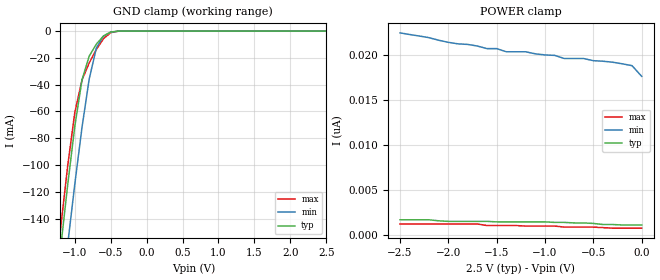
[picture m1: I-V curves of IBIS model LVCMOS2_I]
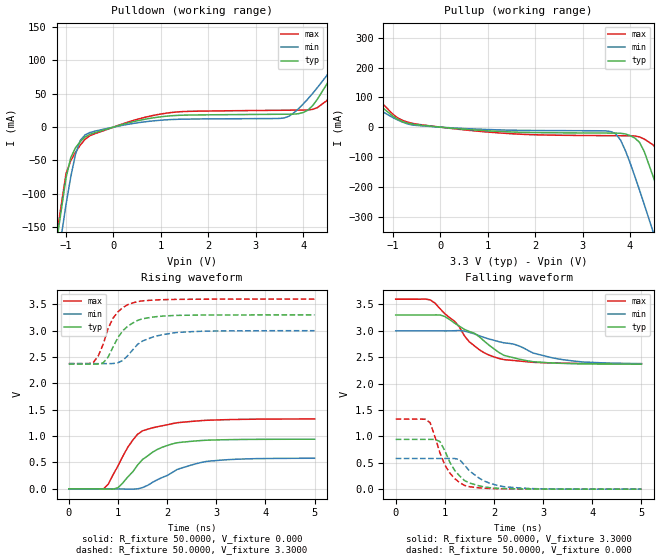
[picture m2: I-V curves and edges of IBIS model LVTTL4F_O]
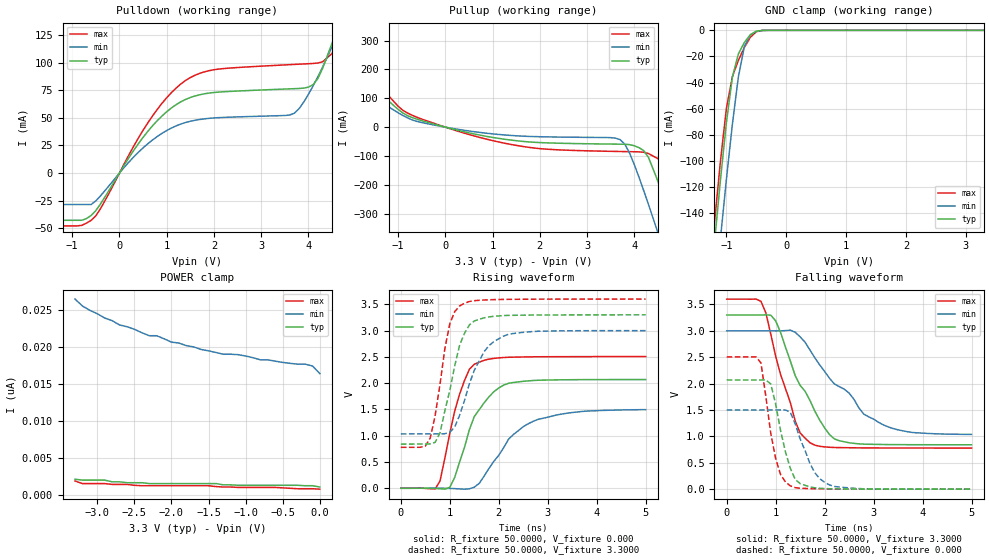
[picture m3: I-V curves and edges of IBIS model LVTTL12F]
| / 7\'7   Xilinx SpartanII I/O Buffer IBIS File
| \ \   Xilinx Inc.
| / /   2100 Logic Drive
| \_\/.\   San Jose,   CA 95124
[IBIS ver]   2.1
[File name]   spartan2.ibs
[File Rev]   1.5
[Date]   Apr. 26, 2002
[Source]   Hspice simulations (23e: TT, SS, FF)
[Notes]   Xilinx IBIS model for SpartanII I/O
   The package models are provided for VQ100, TQ144, CS144,
   PQ208, FG256 and FG456 package types, with VQ100 being
   selected as a default. Please make your own selection of
   the packages by commenting out the unused ones.
   COMMENTS: Models include process corners for MIN and MAX.
[Disclaimer] The data in this model is derived from SPICE simulations using
   modeling information extracted from the target process. While
   a great deal of care has been taken to provide information
   that is accurate, this model is considered preliminary as it
   has not been verified by actual silicon measurement. Treat the
   data in this model as preliminary until actual silicon
   verification is performed.
[Copyright]   Copyright 2000, Xilinx Inc., All rights reserved
|   Component Spartan-II
|   >>> Make Your Selection of the Package type Below <<<
[Component]   Spartan2
[Manufacturer]   Xilinx Inc.
[Package]
|--------------------------- XC2S15 -------------------------------
| XC2S15 with Package type VQ100:
| variable   typ   min   max
R_pkg   89.000m   83.000m   95.000m
L_pkg   4.5500nH   4.0000nH   5.1000nH
C_pkg   0.6500pF   0.6000pF   0.7000pF
| XC2S15 with Package type TQ144:
| variable   typ   min   max
|R_pkg   130.00m   123.00m   137.00m
|L_pkg   8.3500nH   7.5000nH   9.2000nH
|C_pkg   1.0500pF   0.8000pF   1.3000pF
| XC2S15 with Package type CS144:
| variable   typ   min   max
|R_pkg   109.50m   76.000m   143.00m
|L_pkg   2.2500nH   1.5000nH   3.0000nH
|C_pkg   0.2500pF   0.2000pF   0.3000pF
|--------------------------- XC2S30 -------------------------------
| XC2S30 with Package type VQ100:
| variable   typ   min   max
|R_pkg   84.500m   79.000m   90.000m
|L_pkg   4.3500nH   3.8000nH   4.9000nH
|C_pkg   0.6500pF   0.6000pF   0.7000pF
| XC2S30 with Package type TQ144:
| variable   typ   min   max
|R_pkg   130.00m   123.00m   137.00m
|L_pkg   8.3500nH   7.5000nH   9.2000nH
|C_pkg   1.0500pF   0.8000pF   1.3000pF
| XC2S30 with Package type CS144:
| variable   typ   min   max
|R_pkg   109.50m   76.000m   143.00m
|L_pkg   2.2500nH   1.5000nH   3.0000nH
|C_pkg   0.2500pF   0.2000pF   0.3000pF
| XC2S30 with Package type PQ208:
| variable   typ   min   max
|R_pkg   205.50m   205.00m   206.00m
|L_pkg   14.900nH   13.100nH   16.700nH
|C_pkg   1.9000pF   1.7000pF   2.1000pF
|--------------------------- XC2S50 -------------------------------
| XC2S50 with Package type TQ144:
| variable   typ   min   max
|R_pkg   123.50m   117.00m   130.00m
|L_pkg   7.9500nH   7.1000nH   8.8000nH
|C_pkg   1.0000pF   0.8000pF   1.2000pF
| XC2S50 with Package type PQ208:
| variable   typ   min   max
|R_pkg   195.50m   195.00m   196.00m
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[Pin]  signal_name   model_name   R_pin   L_pin   C_pin
1   LVCMOS2   LVCMOS2
1I   LVCMOS2_I   LVCMOS2_I
1O   LVCMOS2_O   LVCMOS2_O
2   LVTTL2F   LVTTL2F
2I   LVTTL2F_I   LVTTL2F_I
2O   LVTTL2F_O   LVTTL2F_O
3   LVTTL4F   LVTTL4F
3I   LVTTL4F_I   LVTTL4F_I
3O   LVTTL4F_O   LVTTL4F_O
4   LVTTL6F   LVTTL6F
4I   LVTTL6F_I   LVTTL6F_I
4O   LVTTL6F_O   LVTTL6F_O
5   LVTTL8F   LVTTL8F
5I   LVTTL8F_I   LVTTL8F_I
5O   LVTTL8F_O   LVTTL8F_O
6   LVTTL12F   LVTTL12F
6I   LVTTL12F_I   LVTTL12F_I
6O   LVTTL12F_O   LVTTL12F_O
7   LVTTL16F   LVTTL16F
7I   LVTTL16F_I   LVTTL16F_I
7O   LVTTL16F_O   LVTTL16F_O
8   LVTTL24F   LVTTL24F
8I   LVTTL24F_I   LVTTL24F_I
8O   LVTTL24F_O   LVTTL24F_O
9   LVTTL2S   LVTTL2S
9I   LVTTL2S_I   LVTTL2S_I
9O   LVTTL2S_O   LVTTL2S_O
10   LVTTL4S   LVTTL4S
10I   LVTTL4S_I   LVTTL4S_I
10O   LVTTL4S_O   LVTTL4S_O
11   LVTTL6S   LVTTL6S
11I   LVTTL6S_I   LVTTL6S_I
11O   LVTTL6S_O   LVTTL6S_O
12   LVTTL8S   LVTTL8S
12I   LVTTL8S_I   LVTTL8S_I
12O   LVTTL8S_O   LVTTL8S_O
13   LVTTL12S   LVTTL12S
13I   LVTTL12S_I   LVTTL12S_I
13O   LVTTL12S_O   LVTTL12S_O
14   LVTTL16S   LVTTL16S
14I   LVTTL16S_I   LVTTL16S_I
14O   LVTTL16S_O   LVTTL16S_O
15   LVTTL24S   LVTTL24S
15I   LVTTL24S_I   LVTTL24S_I
15O   LVTTL24S_O   LVTTL24S_O
16   HSTL1   HSTL1
16I   HSTL1_I   HSTL1_I
16O   HSTL1_O   HSTL1_O
17   HSTL3   HSTL3
17I   HSTL3_I   HSTL3_I
17O   HSTL3_O   HSTL3_O
18   HSTL4   HSTL4
18I   HSTL4_I   HSTL4_I
18O   HSTL4_O   HSTL4_O
19   SSTL2C1   SSTL2C1
19I   SSTL2C1_I   SSTL2C1_I
19O   SSTL2C1_O   SSTL2C1_O
20   SSTL2C2   SSTL2C2
20I   SSTL2C2_I   SSTL2C2_I
20O   SSTL2C2_O   SSTL2C2_O
21   SSTL3C1   SSTL3C1
21I   SSTL3C1_I   SSTL3C1_I
21O   SSTL3C1_O   SSTL3C1_O
22   SSTL3C2   SSTL3C2
22I   SSTL3C2_I   SSTL3C2_I
22O   SSTL3C2_O   SSTL3C2_O
23   CTT   CTT
23I   CTT_I   CTT_I
23O   CTT_O   CTT_O
24   AGP   AGP
24I   AGP_I   AGP_I
24O   AGP_O   AGP_O
25   GTL   GTL
25I   GTL_I   GTL_I
25O   GTL_O   GTL_O
26   GTL-PLUS   GTL-PLUS
26I   GTL-PLUS_I   GTL-PLUS_I
26O   GTL-PLUS_O   GTL-PLUS_O
27   PCI33M5V   PCI33M5V
27I   PCI33M5V_I   PCI33M5V_I
27O   PCI33M5V_O   PCI33M5V_O
28   PCI33M3V   PCI33M3V
28I   PCI33M3V_I   PCI33M3V_I
28O   PCI33M3V_O   PCI33M3V_O
29   PCI66M3V   PCI66M3V
29I   PCI66M3V_I   PCI66M3V_I
29O   PCI66M3V_O   PCI66M3V_O
PGND   GND   GND
VCCO   VCCO   POWER
| Models and submodels in the file (87): LVCMOS2 (I/O), LVCMOS2_I (Input), LVCMOS2_O (Output), LVTTL2F (I/O), LVTTL2F_I (Input), LVTTL2F_O (Output), LVTTL4F (I/O), LVTTL4F_I (Input), LVTTL4F_O (Output), LVTTL6F (I/O), LVTTL6F_I (Input), LVTTL6F_O (Output), LVTTL8F (I/O), LVTTL8F_I (Input), LVTTL8F_O (Output), LVTTL12F (I/O), LVTTL12F_I (Input), LVTTL12F_O (Output), LVTTL16F (I/O), LVTTL16F_I (Input), LVTTL16F_O (Output), LVTTL24F (I/O), LVTTL24F_I (Input), LVTTL24F_O (Output), LVTTL2S (I/O), LVTTL2S_I (Input), LVTTL2S_O (Output), LVTTL4S (I/O), LVTTL4S_I (Input), LVTTL4S_O (Output), LVTTL6S (I/O), LVTTL6S_I (Input), LVTTL6S_O (Output), LVTTL8S (I/O), LVTTL8S_I (Input), LVTTL8S_O (Output), LVTTL12S (I/O), LVTTL12S_I (Input), LVTTL12S_O (Output), LVTTL16S (I/O), LVTTL16S_I (Input), LVTTL16S_O (Output), LVTTL24S (I/O), LVTTL24S_I (Input), LVTTL24S_O (Output), HSTL1 (I/O), HSTL1_I (Input), HSTL1_O (Output), HSTL3 (I/O), HSTL3_I (Input), HSTL3_O (Output), HSTL4 (I/O), HSTL4_I (Input), HSTL4_O (Output), SSTL2C1 (I/O), SSTL2C1_I (Input), SSTL2C1_O (Output), SSTL2C2 (I/O), SSTL2C2_I (Input), SSTL2C2_O (Output), SSTL3C1 (I/O), SSTL3C1_I (Input), SSTL3C1_O (Output), SSTL3C2 (I/O), SSTL3C2_I (Input), SSTL3C2_O (Output), CTT (I/O), CTT_I (Input), CTT_O (Output), AGP (I/O), AGP_I (Input), AGP_O (Output), GTL (I/O_open_drain), GTL_I (Input), GTL_O (Open_drain), GTL-PLUS (I/O_open_drain), GTL-PLUS_I (Input), GTL-PLUS_O (Open_drain), PCI33M5V (I/O), PCI33M5V_I (Input)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
|   Model LVCMOS2_I
[Model]   LVCMOS2_I
Model_type   Input
Polarity   Non-Inverting
Vinl =   0.800V
Vinh =   1.700V
C_comp   6.5000pF   5.0000pF   8.0000pF
[Temperature Range]   27.0000   100.0000   0.000
[Voltage Range]   2.5000V   2.3750V   2.6250V
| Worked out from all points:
|   GND clamp passes 1 mA (typ) near -0.51 V on its own axis
[GND_clamp]
| voltage   I(typ)   I(min)   I(max)
-2.5V     -852.1mA   -861.3mA   -847.6mA
-1.2V     -163.3mA   -206.7mA   -148.3mA
-1.1V     -115.2mA   -159.6mA   -101mA
-1V       -71.03mA   -114.2mA   -60.76mA
-900mV    -36.42mA   -71.86mA   -36.51mA
-800mV    -18.71mA   -35.86mA   -23.83mA
-700mV    -9.708mA   -12.62mA   -13.62mA
-600mV    -3.604mA   -3.647mA   -5.596mA
-500mV    -691.4uA   -852.9uA   -1.154mA
-400mV    -68.33uA   -138.4uA   -98.29uA
2.5V      1.106nA    18.89nA    669.4pA
[POWER_clamp]
| voltage   I(typ)   I(min)   I(max)
-2.5V     1.688nA    22.47nA    1.222nA
-1.7V     1.513nA    21.01nA    1.222nA
-1.6V     1.513nA    20.72nA    1.048nA
-1.5V     1.455nA    20.72nA    1.048nA
-1.4V     1.455nA    20.37nA    1.048nA
-1.2V     1.455nA    20.37nA    989.5pA
-900mV    1.397nA    19.97nA    989.5pA
-800mV    1.397nA    19.62nA    873.1pA
-600mV    1.339nA    19.62nA    873.1pA
-200mV    1.106nA    19.03nA    756.7pA
-100mV    1.106nA    18.83nA    756.7pA
0V        1.106nA    17.64nA    756.7pA
|   Model LVTTL4F_O
[Model]   LVTTL4F_O
Model_type   Output
Polarity   Non-Inverting
Vmeas =   1.4000V
Cref =  35.0000pF
Rref =   1.0000M
Vref =  0.000V
C_comp   6.5000pF   5.0000pF   8.0000pF
[Temperature Range]   27.0000   100.0000   0.000
[Voltage Range]   3.3000V   3.0000V   3.6000V
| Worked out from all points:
|   slope of the pulldown table from 0 to 0.495 V, typ, clamps not added: 52.7 ohm
|   slope of the pullup table from 0 to 0.495 V, typ, clamps not added: 72 ohm
|   rising waveform, R_fixture 50.0000, V_fixture 0.000: 20-80 % time 649ps typ, 853ps min, 538ps max; typ from 0 V to 0.941 V
|   rising waveform, R_fixture 50.0000, V_fixture 3.3000: 20-80 % time 419ps typ, 526ps min, 353ps max; typ from 2.37 V to 3.3 V
|   falling waveform, R_fixture 50.0000, V_fixture 3.3000: 20-80 % time 914ps typ, 1.33ns min, 768ps max; typ from 3.3 V to 2.37 V
|   falling waveform, R_fixture 50.0000, V_fixture 0.000: 20-80 % time 386ps typ, 512ps min, 365ps max; typ from 0.943 V to 0.001 V
[Pulldown]
| voltage   I(typ)   I(min)   I(max)
-3.3V     -1.286A    -1.273A    -1.29A
-1.5V     -317.7mA   -354.1mA   -304.2mA
-1V       -76.21mA   -116mA     -69.81mA
-800mV    -30.95mA   -40.58mA   -37.74mA
-500mV    -10.89mA   -8.192mA   -12.96mA
1.2V      16.95mA    11.33mA    21.76mA
3.6V      19.37mA    13.78mA    25.36mA
4.1V      25.44mA    42.35mA    25.81mA
4.5V      64.6mA     77.61mA    39.82mA
5.1V      143.3mA    138.1mA    128.1mA
5.3V      171mA      159.5mA    161.3mA
6.6V      348mA      295mA      376.7mA
[Pullup]
| voltage   I(typ)   I(min)   I(max)
-3.3V     354.4mA    271.9mA    429.9mA
-2.7V     272.8mA    207.8mA    331mA
-800mV    18.43mA    17.03mA    23.04mA
3.6V      -19.96mA   -15.22mA   -28.65mA
3.8V      -20.52mA   -43.41mA   -28.84mA
4.2V      -51mA      -211.2mA   -32.92mA
4.5V      -171.4mA   -357.8mA   -61.08mA
4.7V      -272mA     -457.9mA   -116mA
4.9V      -376.2mA   -559mA     -210.3mA
5.1V      -482.2mA   -660.7mA   -313.6mA
5.3V      -589.2mA   -762.8mA   -420.3mA
6.6V      -1.293A    -1.432A    -1.133A
[Ramp]
| variable   typ   min   max
dV/dt_r   0.5647/0.6500n   0.3480/0.8497n   0.7950/0.5579n
dV/dt_f   0.5586/0.9517n   0.3726/1.3252n   0.7338/0.7688n
R_load = 50.0000
[Rising Waveform]
R_fixture = 50.0000
V_fixture = 0.000
| time   V(typ)   V(min)   V(max)
0s        0V         0V         0V
700ps     -2.021mV   226.2uV    -4.415mV
800ps     -4.588mV   188uV      85.45mV
1ns       21.52mV    -1.672mV   434.2mV
1.3ns     321.5mV    -6.047mV   921.4mV
1.5ns     557.2mV    23.94mV    1.1V
1.7ns     692mV      121.2mV    1.157V
2.2ns     873.5mV    365.6mV    1.253V
2.8ns     922.2mV    519.7mV    1.3V
5ns       941.2mV    580mV      1.325V
[Rising Waveform]
R_fixture = 50.0000
V_fixture = 3.3000
V_fixture_min = 3.0000
V_fixture_max = 3.6000
| time   V(typ)   V(min)   V(max)
0s        2.365V     2.374V     2.375V
500ps     2.365V     2.374V     2.397V
700ps     2.39V      2.374V     2.744V
800ps     2.499V     2.374V     3.043V
900ps     2.691V     2.377V     3.237V
1.1ns     3V         2.437V     3.439V
1.4ns     3.195V     2.74V      3.551V
1.7ns     3.256V     2.876V     3.579V
2.2ns     3.289V     2.966V     3.594V
5ns       3.299V     2.999V     3.599V
[Falling Waveform]
R_fixture = 50.0000
V_fixture = 3.3000
V_fixture_min = 3.0000
V_fixture_max = 3.6000
| time   V(typ)   V(min)   V(max)
0s        3.3V       3V         3.6V
700ps     3.299V     3V         3.587V
1ns       3.272V     2.999V     3.325V
1.2ns     3.145V     3.002V     3.18V
1.5ns     2.987V     2.97V      2.789V
1.8ns     2.807V     2.874V     2.584V
2.1ns     2.591V     2.795V     2.477V
2.7ns     2.429V     2.625V     2.411V
3.4ns     2.384V     2.454V     2.388V
5ns       2.369V     2.379V     2.377V
[Falling Waveform]
R_fixture = 50.0000
V_fixture = 0.000
| time   V(typ)   V(min)   V(max)
0s        943.3mV    581.6mV    1.327V
600ps     943.4mV    581.6mV    1.325V
700ps     943.7mV    581.6mV    1.262V
900ps     903.3mV    581.6mV    689.3mV
1ns       728.3mV    581.8mV    460.1mV
1.2ns     357.9mV    581.3mV    201.4mV
1.4ns     164mV      456.6mV    71.6mV
1.8ns     43.47mV    155.2mV    18.74mV
2.2ns     11.27mV    47.74mV    7.191mV
5ns       636.3uV    446.4uV    717.8uV
|   Model LVTTL12F
[Model]   LVTTL12F
Model_type   I/O
Polarity   Non-Inverting
Enable   Active-Low
Vinl =   0.800V
Vinh =   2.000V
Vmeas =   1.4000V
Cref =  35.0000pF
Rref =   1.0000M
Vref =  0.000V
C_comp   6.5000pF   5.0000pF   8.0000pF
[Temperature Range]   27.0000   100.0000   0.000
[Voltage Range]   3.3000V   3.0000V   3.6000V
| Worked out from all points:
|   slope of the pulldown table from 0 to 0.495 V, typ, clamps not added: 15.4 ohm
|   slope of the pullup table from 0 to 0.495 V, typ, clamps not added: 25.2 ohm
|   GND clamp passes 1 mA (typ) near -0.51 V on its own axis
|   rising waveform, R_fixture 50.0000, V_fixture 0.000: 20-80 % time 556ps typ, 797ps min, 400ps max; typ from 0 V to 2.07 V
|   rising waveform, R_fixture 50.0000, V_fixture 3.3000: 20-80 % time 372ps typ, 492ps min, 288ps max; typ from 0.84 V to 3.3 V
|   falling waveform, R_fixture 50.0000, V_fixture 3.3000: 20-80 % time 727ps typ, 1.07ns min, 508ps max; typ from 3.3 V to 0.841 V
|   falling waveform, R_fixture 50.0000, V_fixture 0.000: 20-80 % time 305ps typ, 397ps min, 266ps max; typ from 2.07 V to 0 V
[Pulldown]
| voltage   I(typ)   I(min)   I(max)
-3.3V     -42.8mA    -28.54mA   -47.89mA
-900mV    -42.8mA    -28.54mA   -47.89mA
-600mV    -38.47mA   -28.54mA   -42.9mA
700mV     42.79mA    29.97mA    51.76mA
1.2V      61.98mA    42.74mA    77.02mA
1.6V      69.81mA    47.81mA    88.61mA
3.7V      76.41mA    54.11mA    98.37mA
4.1V      80.11mA    79.08mA    99.25mA
4.3V      94.94mA    96.03mA    100.8mA
4.5V      117.6mA    114.4mA    108.3mA
4.7V      142.5mA    133.7mA    132.4mA
6.6V      399mA      330.4mA    441.4mA
[Pullup]
| voltage   I(typ)   I(min)   I(max)
-3.3V     401.3mA    308.2mA    484mA
-2.9V     344.8mA    263.9mA    415.5mA
-2.5V     286.5mA    217.5mA    345.7mA
-700mV    33.24mA    24.98mA    41.08mA
1.5V      -47.01mA   -30.01mA   -63.27mA
3.7V      -59.11mA   -43.28mA   -84.54mA
3.9V      -60.68mA   -90.11mA   -85.1mA
4.2V      -81.62mA   -220.4mA   -87.14mA
4.5V      -188mA     -366.4mA   -109.3mA
4.9V      -390.3mA   -567.4mA   -234.7mA
5.1V      -496.1mA   -669.1mA   -335.2mA
6.6V      -1.307A    -1.441A    -1.153A
[GND_clamp]
| voltage   I(typ)   I(min)   I(max)
-3.3V     -1.286A    -1.273A    -1.29A
-1.3V     -213.2mA   -255.1mA   -198mA
-1.2V     -163mA     -206.8mA   -147.7mA
-1.1V     -114.8mA   -159.6mA   -100.3mA
-1V       -70.57mA   -114.1mA   -59.86mA
-900mV    -35.79mA   -71.75mA   -35.46mA
-800mV    -18.04mA   -35.69mA   -22.98mA
-700mV    -9.256mA   -12.38mA   -13.06mA
-600mV    -3.388mA   -3.468mA   -5.299mA
-500mV    -637.4uA   -792.4uA   -1.07mA
-300mV    -3.973uA   -15.32uA   -4.185uA
3.3V      1.106nA    17.64nA    698.5pA
[POWER_clamp]
| voltage   I(typ)   I(min)   I(max)
-3.3V     2.095nA    26.43nA    1.863nA
-3.2V     1.979nA    25.49nA    1.513nA
-2.9V     1.979nA    23.87nA    1.513nA
-2.3V     1.513nA    21.48nA    1.222nA
-2.2V     1.513nA    21.48nA    1.222nA
-2V       1.513nA    20.61nA    1.222nA
-1.3V     1.339nA    18.98nA    1.048nA
-1.1V     1.281nA    18.92nA    989.5pA
-800mV    1.281nA    18.22nA    989.5pA
-200mV    1.222nA    17.64nA    814.9pA
-100mV    1.222nA    17.4nA     814.9pA
0V        1.048nA    16.36nA    756.7pA
[Ramp]
| variable   typ   min   max
dV/dt_r   1.2408/0.5535n   0.8970/0.7922n   1.5030/0.3954n
dV/dt_f   1.4752/0.7257n   1.1772/1.1183n   1.6925/0.5243n
R_load = 50.0000
[Rising Waveform]
R_fixture = 50.0000
V_fixture = 0.000
| time   V(typ)   V(min)   V(max)
0s        0V         0V         0V
700ps     -3.771mV   692.4uV    -13.4mV
800ps     -9.635mV   799.2uV    138.3mV
1ns       17.96mV    -3.585mV   1.048V
1.2ns     500.5mV    -12.31mV   1.792V
1.5ns     1.364V     21.02mV    2.359V
2ns       1.907V     627.7mV    2.48V
2.2ns     1.998V     933.5mV    2.492V
2.7ns     2.05V      1.273V     2.5V
5ns       2.068V     1.495V     2.505V
[Rising Waveform]
R_fixture = 50.0000
V_fixture = 3.3000
V_fixture_min = 3.0000
V_fixture_max = 3.6000
| time   V(typ)   V(min)   V(max)
0s        840.3mV    1.034V     778.4mV
500ps     841.4mV    1.034V     801.3mV
600ps     844.4mV    1.034V     955.5mV
800ps     1.055V     1.034V     1.98V
1ns       1.861V     1.067V     3.131V
1.2ns     2.721V     1.388V     3.467V
1.4ns     3.108V     1.987V     3.553V
1.7ns     3.242V     2.598V     3.582V
2.1ns     3.285V     2.895V     3.592V
5ns       3.299V     2.998V     3.599V
[Falling Waveform]
R_fixture = 50.0000
V_fixture = 3.3000
V_fixture_min = 3.0000
V_fixture_max = 3.6000
| time   V(typ)   V(min)   V(max)
0s        3.3V       3V         3.6V
700ps     3.299V     3V         3.558V
800ps     3.303V     3V         3.341V
1ns       3.19V      2.999V     2.521V
1.4ns     2.149V     2.973V     1.288V
1.7ns     1.683V     2.638V     880.4mV
2.2ns     952.2mV    1.994V     789.8mV
2.8ns     853.7mV    1.422V     782.3mV
3.2ns     846.6mV    1.218V     780.9mV
5ns       841.4mV    1.038V     779.2mV
[Falling Waveform]
R_fixture = 50.0000
V_fixture = 0.000
| time   V(typ)   V(min)   V(max)
0s        2.07V      1.5V       2.506V
700ps     2.07V      1.5V       2.393V
900ps     1.994V     1.5V       1.06V
1ns       1.615V     1.5V       581mV
1.1ns     1.113V     1.501V     280.2mV
1.3ns     395.3mV    1.458V     63.91mV
1.5ns     105.3mV    953.5mV    17.9mV
1.8ns     26.06mV    311.6mV    8.619mV
2.1ns     8.631mV    80.09mV    4.709mV
5ns       466uV      547.1uV    485uV
